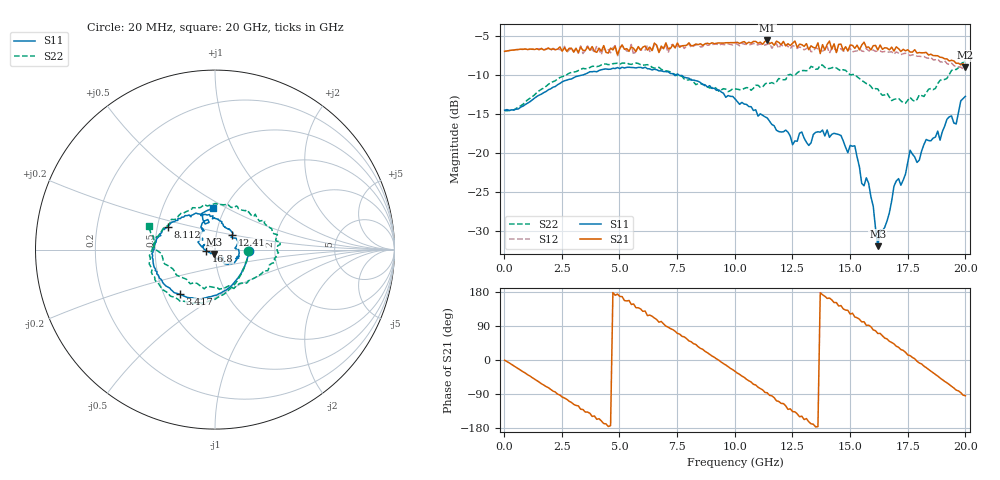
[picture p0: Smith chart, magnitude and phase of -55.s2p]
!Agilent Technologies,N5230A,US43500223,A.07.50.48
!Agilent N5230A: A.07.50.48
!Date: Tuesday, September 15, 2015 18:34:05
!Correction: S11(Full 2 Port(1,2))
!S21(Full 2 Port(1,2))
!S12(Full 2 Port(1,2))
!S22(Full 2 Port(1,2))
!S2P File: Measurements: S11, S21, S12, S22:
# Hz S  dB  R 50
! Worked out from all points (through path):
!   201 points, 20 MHz to 20 GHz, reference 50 ohm
!   highest |S21| = -5.61 dB at 11.41 GHz (marker M1); lowest = -9.0 dB at 20 GHz (marker M2)
!   group delay of S21, straight-line fit = 113 ps
!   lowest |S11| = -32.0 dB at 16.2 GHz (marker M3), VSWR 1.05, Z = 49.3 - j2.42 ohm
!   |S11| at or under -10 dB: start of sweep to 3.443 GHz; 7.364 GHz to 7.467 GHz (102.6 MHz wide, 1.38 % of centre); 7.56 GHz to end of sweep
!   |S22| runs from -14.6 to -8.2 dB; largest |S21 - S12| = 0.098
!   S11 on the Smith chart (normalised r, x): 20 MHz: 1.46, -0.02; 3.417 GHz: 0.61, -0.33; 8.112 GHz: 0.57, +0.16; 12.41 GHz: 1.20, +0.20; 16.8 GHz: 0.91, -0.01; 20 GHz: 0.88, +0.43
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2e7  -14.54 -1.8  -7.00 -0.6  -7.02 -0.6  -14.60 -2.0
1.9181e9  -11.92 -88.0  -6.60 -73.1  -6.56 -74.0  -11.23 -89.1
3.4166e9  -10.03 -128.1  -6.87 -130.7  -7.29 -134.0  -9.18 -124.3
5.1149e9  -9.04 -160.7  -6.17 167.3  -6.35 164.6  -8.52 -157.7
6.7133e9  -9.50 174.3  -7.16 99.8  -7.07 97.9  -9.05 175.8
8.1119e9  -10.69 154.2  -6.31 48.2  -6.53 43.4  -10.59 145.2
9.011e9  -11.75 138.1  -5.91 10.5  -6.13 8.6  -11.69 119.6
1.001e10  -13.09 115.8  -5.89 -29.9  -5.99 -33.2  -11.81 88.6
1.14086e10  -15.54 83.9  -5.61 -86.5  -6.11 -91.9  -11.01 51.8
1.24076e10  -17.87 40.5  -6.27 -128.8  -6.68 -133.9  -9.94 29.8
1.34066e10  -17.65 1.3  -6.51 -169.6  -7.02 -172.4  -9.06 11.8
1.41059e10  -18.02 -23.6  -5.70 163.4  -7.24 157.5  -9.20 -0.8
1.52048e10  -19.10 -47.9  -6.62 113.6  -6.98 112.4  -9.99 -21.8
1.55045e10  -23.91 -46.7  -6.20 100.7  -6.96 99.0  -10.72 -27.5
1.58042e10  -23.90 -59.7  -6.45 91.9  -6.93 86.3  -11.19 -33.7
1.62038e10  -31.95 -104.2  -6.83 70.1  -6.98 69.5  -11.82 -46.7
1.67033e10  -27.68 -163.9  -6.82 49.3  -7.10 47.6  -12.86 -66.2
1.68032e10  -26.17 -173.8  -6.47 46.3  -7.06 43.2  -13.31 -68.9
1.76024e10  -19.67 156.2  -7.09 11.6  -7.55 8.5  -12.89 -105.2
1.83017e10  -18.29 131.4  -7.14 -20.1  -7.83 -23.3  -12.33 -140.5
1.96004e10  -16.30 111.1  -8.54 -79.5  -9.01 -80.2  -9.34 172.2
2e10  -12.77 92.7  -9.05 -94.3  -9.33 -98.9  -8.24 160.5
